ORGANIZATION_BLOCK MAIN:OB1
TITLE= Marcia/Arresto M.A.T.
// Simulatore: 00
// Versione: 1.0
// Data: 26/02/2002
//-------------------- Descrizione Programma ---------------
// Gestione di un Marcia/Arresto completo di segnalazioni
// mediante istruzioni di SET RESET e Fronte di Discesa del
// contatto ausiliario di KM per il reset delle uscite.
//
// Come prescritto dalle norme il relè termico FR dovrà
// intervenire direttamente in hardware alla diseccitazione del
// contattore KM; l'informazione dell'intervento viene portata al
// PLC mediante un ulteriore contatto del relè al fine di
// permettere al programma di disattivare le uscite e segnalarne
// l'intervento con la lampada gestita dall'uscita Q0.3.
// Il programma grazie all'interrogazione sul fronte di discesa del
// contatto ausiliario di KM provvederà a resettare l'uscita anche
// quando per cause esterne (circuiti di sicurezza, intervento termico)
// il contattore KM viene diseccitato.

BEGIN
NETWORK 1 //Set KM Linea
//
LD I0.1
A I0.3
A I0.0
S Q0.0 1

NETWORK 2 //Reset KM Linea
//
LD I0.2
ED
ON I0.3
ON I0.0
R Q0.0 1

NETWORK 3 //Segnalazione Marcia
//
LD Q0.0
= Q0.2

NETWORK 4 //Segnalazione Arresto
//
LDN Q0.0
= Q0.1

NETWORK 5 //Segnalazione Relè termico scattato
//
LDN I0.3
= Q0.3

END_ORGANIZATION_BLOCK

